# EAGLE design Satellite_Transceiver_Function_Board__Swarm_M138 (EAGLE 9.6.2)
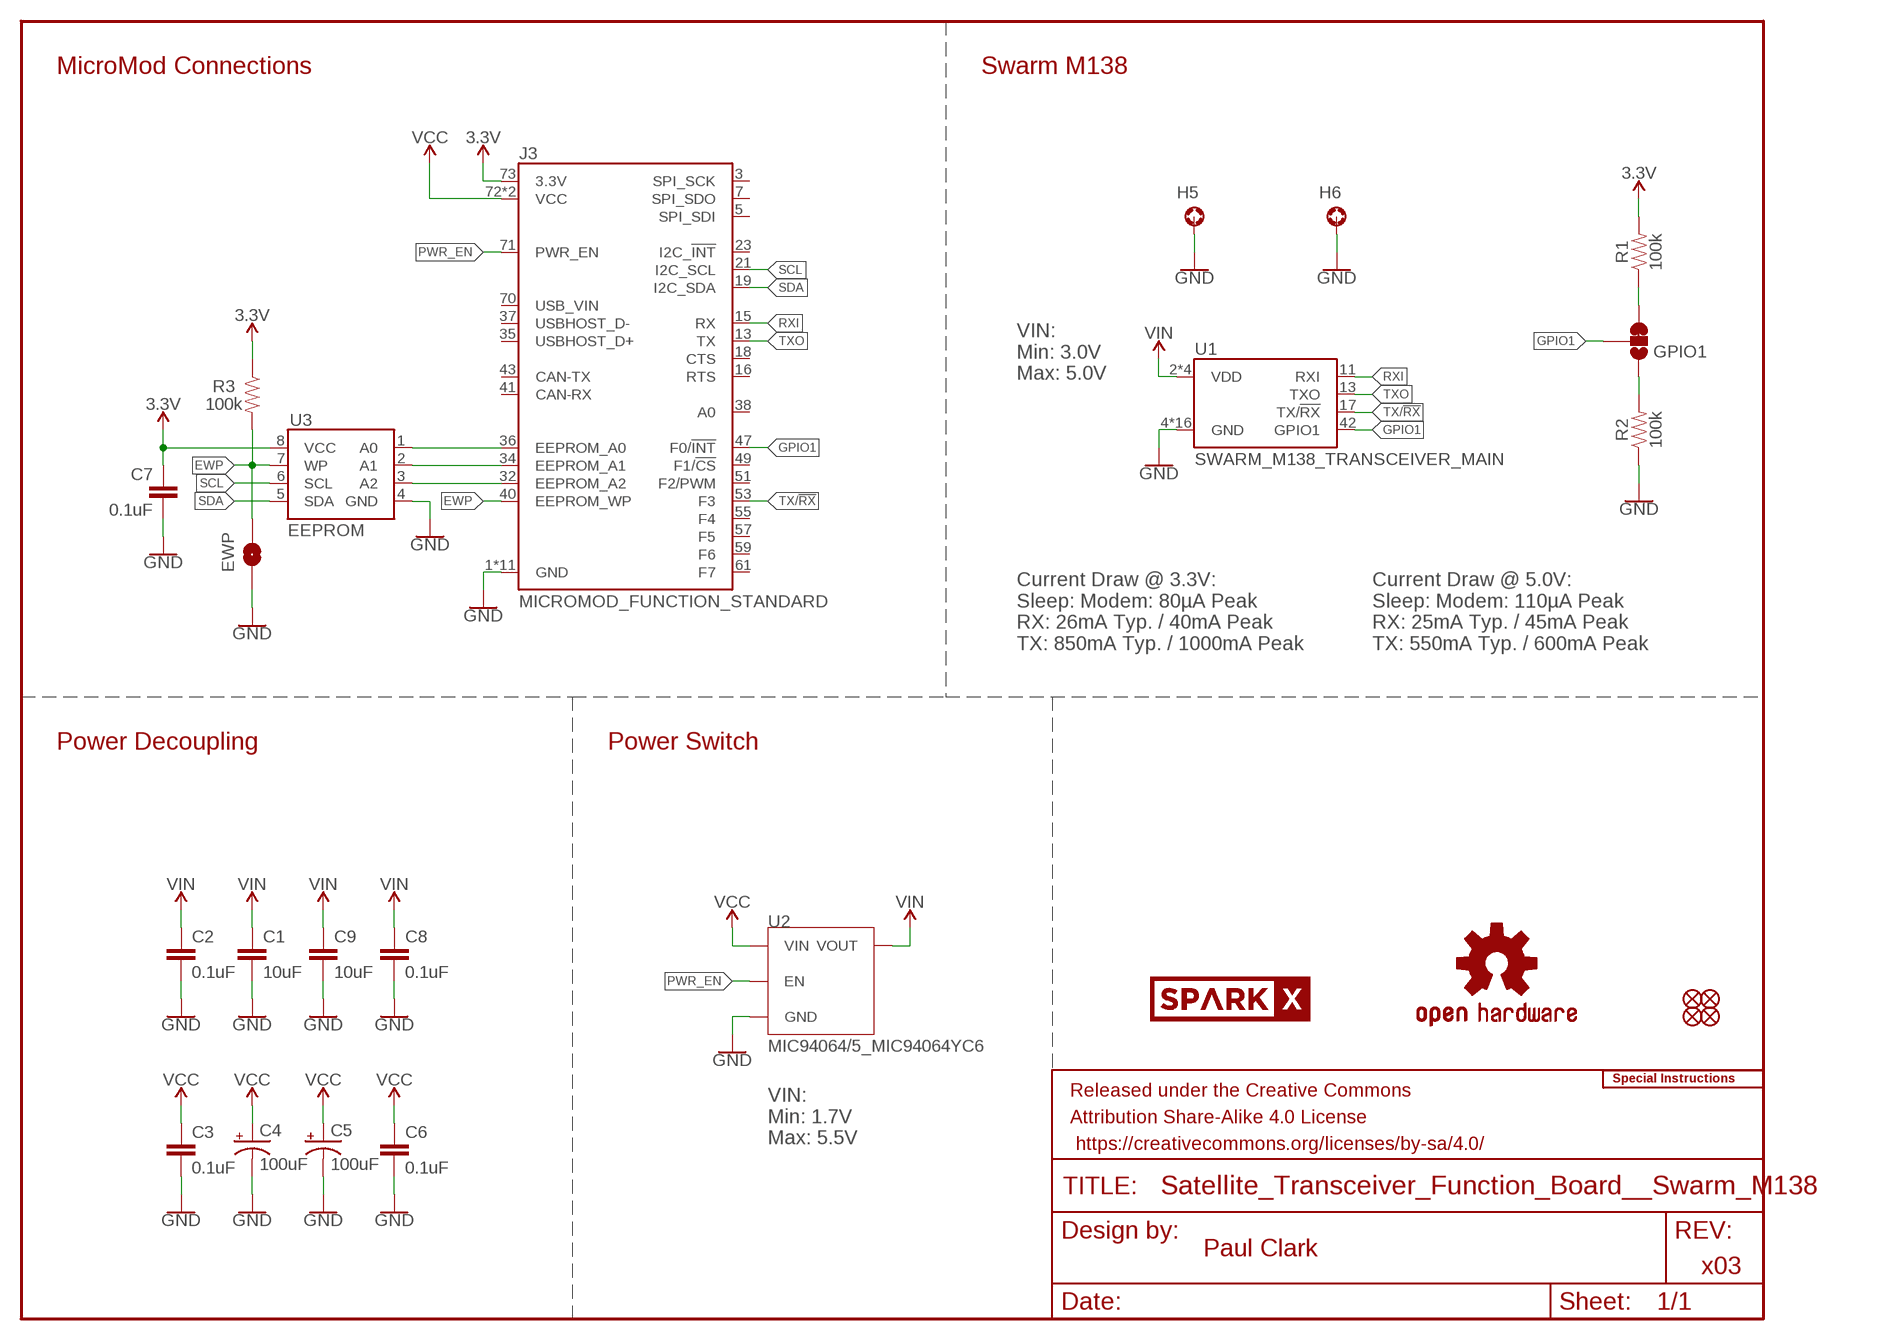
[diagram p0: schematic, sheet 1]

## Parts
C1  10uF  10UF-0603-6.3V-20%  [0603]
C2  0.1uF  0.1UF-0603-25V-5%  [0603]
C3  0.1uF  0.1UF-0603-25V-5%  [0603]
C4  100uF  100UF-POLAR-EIA3528-10V-20%(TANT)  [EIA3528]
C5  100uF  100UF-POLAR-EIA3528-10V-20%(TANT)  [EIA3528]
C6  0.1uF  0.1UF-0603-25V-5%  [0603]
C7  0.1uF  0.1UF-0603-25V-5%  [0603]
C8  0.1uF  0.1UF-0603-25V-5%  [0603]
C9  10uF  10UF-0603-6.3V-20%  [0603]
EWP  JUMPER-SMT_2_NO_SILK  [SMT-JUMPER_2_NO_SILK]
FD1  FIDUCIAL1X2  [FIDUCIAL-1X2]
FD2  FIDUCIAL1X2  [FIDUCIAL-1X2]
FD3  FIDUCIAL1X2  [FIDUCIAL-1X2]
FD4  FIDUCIAL1X2  [FIDUCIAL-1X2]
FRAME1  FRAME-LETTER  [CREATIVE_COMMONS]
GPIO1  JUMPER-SMT_3_1-NC_TRACE_SILK  [SMT-JUMPER_3_1-NC_TRACE_SILK]
H5  STAND-OFF-REFLOW-M2.5_1.5MM_TALL  [STAND-OFF-REFLOW-M2.5]
H6  STAND-OFF-REFLOW-M2.5_1.5MM_TALL  [STAND-OFF-REFLOW-M2.5]
J3  MICROMOD_FUNCTION_STANDARD  [M.2-CARD-E-22_FUNCTION_STANDARD]
LOGO1  SPECIAL_INSTRUCTIONS-ORDERING  [ORDERING_INSTRUCTIONS]
LOGO2  OSHW-LOGOM  [OSHW-LOGO-M]
LOGO3  OSHW-LOGOM  [OSHW-LOGO-M]
R1  100k  100KOHM-0603-1/10W-1%  [0603]
R2  100k  100KOHM-0603-1/10W-1%  [0603]
R3  100k  100KOHM-0603-1/10W-1%  [0603]
U1  SWARM_M138_TRANSCEIVER_MAIN  [M.2-SWARM-M138-A]
U2  MIC94064/5_MIC94064YC6  [SC-70-6]
U3  EEPROM  EEPROM-I2C512K  [SO08]
U$1  SPARKX-LOGO5  [SPARKX-LARGE]
U$2  SPARKX-LOGO5  [SPARKX-LARGE]

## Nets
3.3V: C7.1 J3.73(3.3V) R1.2 R3.1 U3.8(VCC)
A0 [DIGITAL]: J3.36(EEPROM_A0) U3.1(A0)
A1 [DIGITAL]: J3.34(EEPROM_A1) U3.2(A1)
A2 [DIGITAL]: J3.32(EEPROM_A2) U3.3(A2)
EWP [DIGITAL]: EWP.2 J3.40(EEPROM_WP) R3.2 U3.7(WP)
GND: C1.2 C2.2 C3.2 C4.C(-) C5.C(-) C6.2 C7.2 C8.2 C9.2 EWP.1 H5.1 H6.1 J3.1(GND) J3.33(GND) J3.39(GND) J3.45(GND) J3.75(GND) J3.GND1(GND) J3.GND2(GND) J3.GND3(GND) J3.GND4(GND) J3.GND5(GND) J3.GND6(GND) R2.1 U1.4(GND) U1.9(GND) U1.15(GND) U1.18(GND) U1.21(GND) U1.26(GND) U1.27(GND) U1.29(GND) U1.34(GND) U1.35(GND) U1.37(GND) U1.40(GND) U1.43(GND) U1.50(GND) U1.A1(GND) U1.A2(GND) U2.2(GND) U2.5(GND) U3.4(GND)
GPIO1: GPIO1.2 J3.47(F0/!INT!) U1.42(GPIO1)
N$14: GPIO1.3 R1.1
N$16: GPIO1.1 R2.2
PWR_EN: J3.71(PWR_EN) U2.3(EN)
RXI: J3.15(RX) U1.11(RXI)
SCL [DIGITAL]: J3.21(I2C_SCL) U3.6(SCL)
SDA [DIGITAL]: J3.19(I2C_SDA) U3.5(SDA)
TX/!RX!: J3.53(F3) U1.17(TX/!RX!)
TXO: J3.13(TX) U1.13(TXO)
VCC: C3.1 C4.A(+) C5.A(+) C6.1 J3.72(VCC) J3.74(VCC) U2.4(VIN)
VIN: C1.1 C2.1 C8.1 C9.1 U1.2(VDD) U1.39(VDD) U1.41(VDD) U1.52(VDD) U2.1(VOUT)
Unconnected: J3.3(SPI_SCK) J3.5(SPI_SDI) J3.7(SPI_SDO) J3.16(RTS) J3.18(CTS) J3.23(I2C_!INT!) J3.35(USBHOST_D+) J3.37(USBHOST_D-) J3.38(A0) J3.41(CAN-RX) J3.43(CAN-TX) J3.49(F1/!CS!) J3.51(F2/PWM) J3.55(F4) J3.57(F5) J3.59(F6) J3.61(F7) J3.70(USB_VIN)

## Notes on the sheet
- MicroMod Connections | Swarm M138
- VIN:
  Min: 3.0V
  Max: 5.0V
- Current Draw @ 3.3V:
  Sleep: Modem: 80µA Peak
  RX: 26mA Typ. / 40mA Peak
  TX: 850mA Typ. / 1000mA Peak
- Current Draw @ 5.0V:
  Sleep: Modem: 110µA Peak
  RX: 25mA Typ. / 45mA Peak
  TX: 550mA Typ. / 600mA Peak
- Power Decoupling | Power Switch
- VIN:
  Min: 1.7V
  Max: 5.5V
- Paul Clark
- x03

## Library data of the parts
C1 C9 = SparkFun-Capacitors:10UF: 10.0µF ceramic capacitors; PROD_ID: CAP-11015
C2 C3 C6-C8 = SparkFun-Capacitors:0.1UF: 0.1µF ceramic capacitors; PROD_ID: CAP-08604
C4 C5 = SparkFun-Capacitors:100UF-POLAR: 100µF polarized capacitors; PROD_ID: CAP-16823
EWP = SparkFun-Jumpers:JUMPER-SMT_2_NO: Normally open jumper
FD1-FD4 = SparkFun-Aesthetics:FIDUCIAL: Fiducial Alignment Points
FRAME1 = SparkFun-Aesthetics:FRAME-LETTER: Schematic Frame - Letter
GPIO1 = SparkFun-Jumpers:JUMPER-SMT_3_1-NC_TRACE: Normally closed trace jumper (1 of 2 connections) This jumper has a trace between two pads so it's normally closed (NC). The other connection is normally open (NO). Use a razor knife to open the connection. For best results follow the IPC guidelines for cutting traces: Cutout at least 0.063 mm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
H5 H6 = SparkFun-Hardware:STAND-OFF-REFLOW: Stand Off Reflow Compatible; PROD_ID: HW-16629
J3 = SparkFun-MicroMod:MICROMOD_FUNCTION: MicroMod Connector Description: A card edge connector and mating PCB connector to allow various MicroMod Processor Boards to be coupled with various carrier boards of different capabilities. Based on the M.2 standard.
LOGO1 = SparkFun-Aesthetics:SPECIAL_INSTRUCTIONS: Special Ordering/Production Instructions Alert
LOGO2 LOGO3 = SparkFun-Aesthetics:OSHW-LOGO: Open-Source Hardware (OSHW) Logo
R1-R3 = SparkFun-Resistors:100KOHM: 100kΩ resistor; PROD_ID: RES-07828
U1 = SparkFun-RF:SWARM_M138_TRANSCEIVER: Swarm M138 Modem Description: A satellite transceiver based on the mPCIe standard.; PROD_ID: CONN-16558
U2 = SparkFun-IC-Power:MIC94064/5: The MIC94064 and MIC94065 are high-side load switches designed for operation between 1.7V to 5.5V. The devices contain a low on-resistance P-channel MOSFET that supports over 2A of continuous current. The MIC94064/5 provides a slew rate controlled SoftStart turn-on of 115µs (typical) to prevent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; PROD_ID: IC-16794
U3 = SparkFun-IC-Memory:EEPROM-I2C: I2C EEPROMs, 24LC256 and others 24LC256 Series 256 kb I2C 2 Wire (32 k x 8 Bit) 2.5 V Serial EEPROM SMD - SOIC-8 Datasheet SparkFun Products SparkFun UDB5 - PIC UAV Development Board (GPS-11703); PROD_ID: IC-14645
U$1 U$2 = SparkX:SPARKX-LOGO

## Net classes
4 3.3V: width 0.2 mm, clearance 0.2 mm to class 1
10 DIGITAL: width 0.09 mm, clearance 0.1 mm to class 0, clearance 0.1 mm to class 1, clearance 0.1 mm

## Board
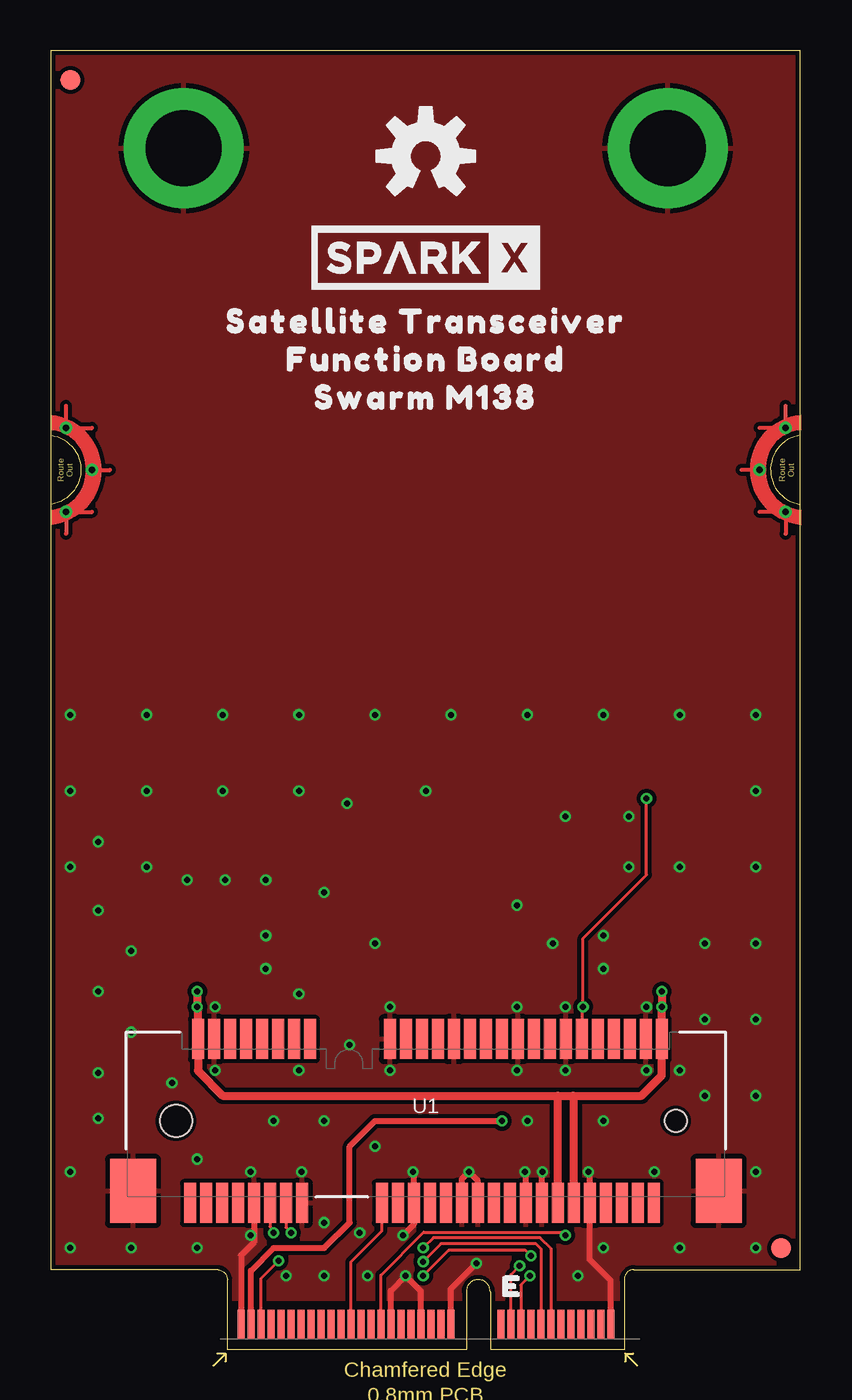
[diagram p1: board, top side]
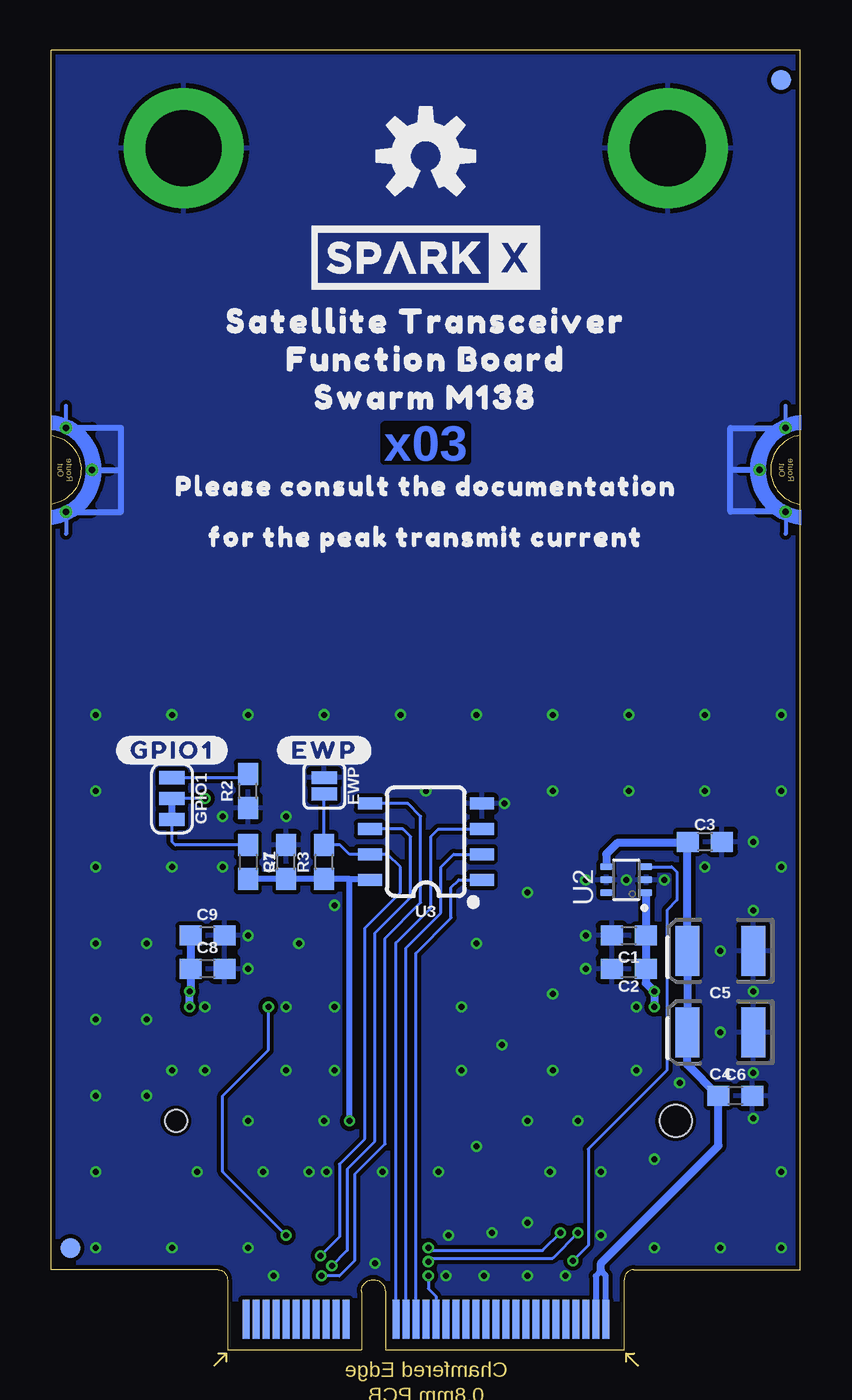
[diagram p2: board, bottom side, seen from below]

Size 37.5 x 65 mm. Coordinates in mm from the lower left corner, seen from the top.
Outline: 28.67,0 21.97,0 21.97,2.9 arc180 20.77,2.9 20.77,0 8.82,0 8.82,3.5 arc84 8.35,4 0,4 0,65 37.49,65 37.49,4 29.15,4 arc85 28.67,3.5 28.67,0
Copper layers (1*16): Top 0.035mm / dielectric 1.5mm / Bottom 0.035mm
Design rules "SparkFun-2-Layer-Minimum-JLCPCB": minimum track width 5mil, minimum drill 0.3mm, track to track 5mil, track to pad 5mil, pad to pad 5mil, via to via 5mil, smd to smd 5mil, copper to edge 7mil, drill to drill 7mil, minimum pad ring 5mil, minimum via ring 5mil, stop-mask expansion 2.5mil, vias tented up to drill 25mil, thermal gap 10mil
tRestrict: 2 lines

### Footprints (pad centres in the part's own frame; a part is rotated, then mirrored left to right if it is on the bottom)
0603 = smd 1.1 x 1: 1 -0.85,0; 2 0.85,0
EIA3528 = smd 1.2 x 2.5: A 1.65,0; C -1.65,0
SMT-JUMPER_2_NO_SILK = smd 0.635 x 1.27: 1 -0.406,0; 2 0.406,0
FIDUCIAL-1X2 = smd 1 x 1: 1 0,0
SMT-JUMPER_3_1-NC_TRACE_SILK = smd 0.66 x 1.27: 1 -1.041,0; 2 0,0; 3 1.041,0
STAND-OFF-REFLOW-M2.5 = drill 3.8 pad 6: 1 0,0
M.2-CARD-E-22_FUNCTION_STANDARD = smd 0.35 x 1.45: 1 9.25,1.275; 3 8.75,1.275; 5 8.25,1.275; 7 7.75,1.275; 9 7.25,1.275; 11 6.75,1.275; 13 6.25,1.275; 15 5.75,1.275; 17 5.25,1.275; 19 4.75,1.275; 21 4.25,1.275; 23 3.75,1.275; 33 1.25,1.275; 35 0.75,1.275; 37 0.25,1.275; 39 -0.25,1.275; 41 -0.75,1.275; 43 -1.25,1.275; 45 -1.75,1.275; 47 -2.25,1.275; 49 -2.75,1.275; 51 -3.25,1.275; 53 -3.75,1.275; 55 -4.25,1.275; 57 -4.75,1.275; 59 -5.25,1.275; 61 -5.75,1.275; 63 -6.25,1.275; 65 -6.75,1.275; 67 -7.25,1.275; 69 -7.75,1.275; 71 -8.25,1.275; 73 -8.75,1.275; 75 -9.25,1.275 | smd 0.35 x 1.95 bottom: 2 9,1.525; 4 8.5,1.525; 6 8,1.525; 8 7.5,1.525; 10 7,1.525; 12 6.5,1.525; 14 6,1.525; 16 5.5,1.525; 18 5,1.525; 20 4.5,1.525; 22 4,1.525; 32 1.5,1.525; 34 1,1.525; 36 0.5,1.525; 38 0,1.525; 40 -0.5,1.525; 42 -1,1.525; 44 -1.5,1.525; 46 -2,1.525; 48 -2.5,1.525; 50 -3,1.525; 52 -3.5,1.525; 54 -4,1.525; 56 -4.5,1.525; 58 -5,1.525; 60 -5.5,1.525; 62 -6,1.525; 64 -6.5,1.525; 66 -7,1.525; 68 -7.5,1.525; 70 -8,1.525; 72 -8.5,1.525; 74 -9,1.525 | drill 0.305 pad 0.61: GND1 -18,41.9; GND2 -16.7,44; GND3 -18,46.1; GND4 18,41.9; GND5 16.7,44; GND6 18,46.1
M.2-SWARM-M138-A = smd 0.6 x 2: 1 -11.8,-4.1; 2 -11.4,4.1; 3 -11,-4.1; 4 -10.6,4.1; 5 -10.2,-4.1; 6 -9.8,4.1; 7 -9.4,-4.1; 8 -9,4.1; 9 -8.6,-4.1; 10 -8.2,4.1; 11 -7.8,-4.1; 12 -7.4,4.1; 13 -7,-4.1; 14 -6.6,4.1; 15 -6.2,-4.1; 16 -5.8,4.1; 17 -2.2,-4.1; 18 -1.8,4.1; 19 -1.4,-4.1; 20 -1,4.1; 21 -0.6,-4.1; 22 -0.2,4.1; 23 0.2,-4.1; 24 0.6,4.1; 25 1,-4.1; 26 1.4,4.1; 27 1.8,-4.1; 28 2.2,4.1; 29 2.6,-4.1; 30 3,4.1; 31 3.4,-4.1; 32 3.8,4.1; 33 4.2,-4.1; 34 4.6,4.1; 35 5,-4.1; 36 5.4,4.1; 37 5.8,-4.1; 38 6.2,4.1; 39 6.6,-4.1; 40 7,4.1; 41 7.4,-4.1; 42 7.8,4.1; 43 8.2,-4.1; 44 8.6,4.1; 45 9,-4.1; 46 9.4,4.1; 47 9.8,-4.1; 48 10.2,4.1; 49 10.6,-4.1; 50 11,4.1; 51 11.4,-4.1; 52 11.8,4.1 | smd 2.3 x 3.2: A1 -14.65,-3.5; A2 14.65,-3.5 | hole 1.1: 12.5,0 | hole 1.6: -12.5,0
SC-70-6 = smd 0.35 x 0.6: 1 -0.65,-1; 2 0,-1; 3 0.65,-1; 4 0.65,1; 5 0,1; 6 -0.65,1
SO08 = smd 0.6 x 1.2: 1 -1.905,-2.8; 2 -0.635,-2.8; 3 0.635,-2.8; 4 1.905,-2.8; 5 1.905,2.8; 6 0.635,2.8; 7 -0.635,2.8; 8 -1.905,2.8

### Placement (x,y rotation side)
C1  8.59,20.7 180 bottom
C2  8.59,19.05 180 bottom
C3  4.78,25.4 0 bottom
C4  4.02,15.88 180 bottom
C5  4.02,19.94 180 bottom
C6  3.25,12.7 0 bottom
C7  25.73,24.38 90 bottom
C8  29.67,19.05 0 bottom
C9  29.67,20.7 0 bottom
EWP  23.83,28.19 270 bottom
FD1  36.53,5.08 0 top
FD2  36.53,5.08 0 bottom
FD3  0.97,63.5 0 top
FD4  0.97,63.5 0 bottom
FRAME1  not placed on the board
GPIO1  31.45,27.56 270 bottom
H5  6.65,60.08 0 top
H6  30.85,60.08 0 top
J3  18.75,0 0 top
LOGO1  not placed on the board
LOGO2  18.75,59.69 0 top
LOGO3  18.75,59.69 0 bottom
R1  27.64,24.38 270 bottom
R2  27.64,27.94 90 bottom
R3  23.83,24.38 90 bottom
U1  18.75,11.43 0 top
U2  8.71,23.5 90 bottom
U3  18.75,25.4 90 bottom
U$1  18.75,54.61 0 bottom
U$2  18.75,54.61 0 top
U$3  [FUNCTION_BOARD0]  18.75,49.53 0 top
U$4  [SATELLITE_TRANSCEIVER0]  18.75,51.44 0 top
U$5  [SATELLITE_TRANSCEIVER0]  18.75,51.44 0 bottom
U$6  [PLEASE_CONSULT_THE_DOCUMENTATION0]  18.75,43.18 0 bottom
U$7  [FUNCTION_BOARD0]  18.75,49.53 0 bottom
U$8  [#EWP#0]  23.83,29.97 0 bottom
U$19  [#GPIO1#0]  31.45,29.97 0 bottom
U$31  [FOR_THE_PEAK_TRANSMIT_CURRENT1]  18.75,40.64 0 bottom
U$40  [SWARM_M1381]  18.75,47.62 0 top
U$41  [SWARM_M1381]  18.75,47.62 0 bottom

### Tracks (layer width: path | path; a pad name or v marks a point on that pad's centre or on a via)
3.3V  (via drill 0.3)
  Top 0.305: J3.73 10,3.95 11.13,5.08 13.67,5.08 14.94,6.35 14.94,10.16 16.21,11.43 v22.56,11.43
  Bottom 0.305: v22.56,11.43 22.56,23.53 | 22.56,23.53 R3.1 C7.1 R1.2 | 22.56,23.53 21.59,23.53 U3.8
A0
  Bottom 0.152: U3.1 17.1,23.5 17.48,23.11 17.48,21.59 19.25,19.82 J3.36
A1
  Bottom 0.152: U3.2 17.35,24.77 17.98,24.13 17.98,21.84 19.75,20.08 J3.34
A2
  Bottom 0.152: J3.32 20.25,20.34 18.49,22.1 18.49,25.65 18.11,26.04 U3.3
EWP  (via drill 0.3)
  Top 0.152: v24.02,4.68 23.75,4.95 19.89,4.95 v18.62,3.68
  Bottom 0.152: v24.02,4.68 23.06,5.63 23.06,9.27 21.8,10.54 21.8,21.08 20.02,22.86 20.02,24.13 20.65,24.77 U3.7 22.56,24.77 23.03,25.23 R3.2 EWP.2 | v18.62,3.68 18.62,3.05 18.25,2.67 J3.40
GND  (via drill 0.3)
  Top 0.305: J3.1 28,3.45 26.95,4.5 U1.43 26.95,8.82 v26.88,8.89 | U1.9 10.15,5.37 9.5,4.72 J3.75 | J3.33 20,3.03 v21.29,4.32 | U1.27 20.55,8.53 v20.91,8.89 21.35,8.45 U1.29 | v18.11,8.89 18.15,8.86 U1.21 18.15,6.26 v17.6,5.71 | U1.35 23.75,8.84 v23.7,8.89 | U1.37 24.55,8.85 v24.59,8.89 | J3.39 18.5,2.92 v17.73,3.68 17,2.95 J3.45
  Bottom 0.305: J3.GND1 3.51,41.91 3.51,44 | J3.GND3 3.51,46.1 3.51,44 | J3.GND2 3.51,44 | J3.GND5 33.99,44 | J3.GND6 33.99,46.1 33.99,44 | J3.GND4 33.99,41.9 33.99,44
  other vias: 16.97,13.97 23.32,13.97 25.73,13.97 29.8,13.97 2.36,25.4 9.98,8.89 8.21,13.97 12.52,8.89 27.64,19.05 25.73,17.14 23.32,17.14 16.97,17.14 29.8,17.14 31.45,13.97 27.64,11.43 16.21,10.16 13.67,11.43 13.67,6.35 15.45,5.84 13.67,3.68 26.37,3.68 7.32,5.08 0.97,5.08 2.36,17.91 2.36,21.97 0.97,31.75 4.78,31.75 8.59,31.75 12.4,31.75 16.21,31.75 20.02,31.75 23.83,31.75 35.26,31.75 8.59,27.94 12.4,27.94 31.45,31.75 35.26,24.13 27.64,31.75 8.21,17.14 12.4,17.78 12.4,13.97 2.36,13.84 11.13,11.43 30.18,8.89 31.45,5.08 35.26,27.94 2.36,11.56 4.02,5.08 15.83,3.68 9.98,5.71 23.83,11.43 11.76,3.68 35.26,5.08 8.71,23.5 6.81,23.5 10.75,23.5 7.32,9.53 6.05,13.34 0.97,8.89 4.02,19.94 4.02,15.88 10.75,20.7 10.75,19.05 4.78,27.94 0.97,27.94 27.64,20.7 14.81,27.3 25.73,26.67 0.97,24.13 4.78,24.13 31.45,24.13 35.26,20.32 35.26,16.51 35.26,12.7 35.26,8.89 32.72,20.32 32.72,16.51 32.72,12.7 25.1,20.32 16.21,20.32 14.94,15.24 13.67,22.86 23.32,22.23 18.75,27.94 27.64,5.08 28.91,24.13 28.91,26.67
  pour Top (isolate 0.203): -0.3,2.54 -0.3,66.04 37.8,66.04 37.8,2.54
  pour Bottom (isolate 0.203): -0.3,2.54 -0.3,66.04 37.8,66.04 37.8,2.54
GPIO1  (via drill 0.3)
  Top 0.152: J3.47 16.5,3.72 18.64,5.87 25.58,5.87 v25.73,5.71 | U1.42 26.55,17.07 v26.62,17.14 26.62,20.57 29.8,23.75 v29.8,27.56
  Bottom 0.152: v25.73,5.71 28.91,8.89 28.91,12.7 26.62,14.99 v26.62,17.14 | v29.8,27.56 GPIO1.2
N$14
  Bottom 0.152: R1.1 31.28,25.23 31.45,25.4 GPIO1.3
N$16
  Bottom 0.152: GPIO1.1 27.83,28.6 R2.2
PWR_EN  (via drill 0.3)
  Top 0.152: J3.71 10.5,3.56 v11.38,4.45
  Bottom 0.152: U2.3 6.44,24.14 6.17,23.88 6.17,22.48 6.68,21.97 6.68,13.97 10.62,10.03 10.62,5.21 v11.38,4.45
RXI  (via drill 0.3)
  Top 0.152: U1.11 10.95,6.15 11.13,5.97 v11.13,5.84 | v18.62,4.4 19.51,5.29 24.25,5.29 24.5,5.04 J3.15
  Bottom 0.152: v11.13,5.84 12.4,4.57 18.45,4.57 v18.62,4.4
SCL  (via drill 0.3)
  Top 0.152: J3.21 23,3.74 v23.45,4.19
  Bottom 0.152: v23.45,4.19 22.68,4.95 22.68,9.02 21.29,10.41 21.29,20.83 19.51,22.61 19.51,25.65 19.89,26.04 U3.6
SDA  (via drill 0.3)
  Top 0.152: v23.95,3.68 23.5,3.23 J3.19
  Bottom 0.152: v23.95,3.68 23.06,3.68 22.3,4.45 22.3,8.76 20.78,10.29 20.78,20.57 19,22.35 19,26.67 19.64,27.3 U3.5
TX/!RX!
  Top 0.152: J3.53 15,4.38 16.55,5.93 U1.17
TXO  (via drill 0.3)
  Top 0.152: U1.13 11.75,6.11 v12.02,5.84 | J3.13 25,5.05 24.46,5.59 19.13,5.59 v18.62,5.08
  Bottom 0.152: v18.62,5.08 18.49,4.95 12.91,4.95 v12.02,5.84
VCC
  Bottom 0.305: J3.74 9.75,3.7 9.98,3.94 10.25,3.67 J3.72 | 9.71,24.24 U2.4
  Bottom 0.406: 9.98,3.94 9.98,4.32 4.1,10.2 C6.1 5.66,14.26 C4.A C5.A 5.66,25.36 | 9.71,24.24 9.71,24.78 9.13,25.36 5.66,25.36 | 5.66,25.36 C3.1
VIN  (via drill 0.3)
  Top 0.406: 25.35,12.7 8.59,12.7 7.35,13.94 U1.2 7.35,17.11 v7.32,17.14 v7.32,17.91 | 25.35,12.7 26.11,12.7 | 26.11,12.7 29.54,12.7 30.55,13.71 U1.52 v30.55,17.13 v30.56,17.14 v30.56,17.91 | U1.39 25.35,12.7 | U1.41 26.15,12.67 26.11,12.7
  Bottom 0.305: 7.71,22.62 U2.1
  Bottom 0.406: v7.32,17.14 v7.32,17.91 7.74,18.33 C2.1 C1.1 7.71,20.72 7.71,22.62 | v30.56,17.14 v30.56,17.91 30.52,17.95 C8.1 C9.1

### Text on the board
Bottom: x03
Measures: Dimensions in mm
tDocu: 2-Layer Board / 0.8mm Thickness / 1oz Copper / ENIG Finish / Chamfered Edge | Paul Clark

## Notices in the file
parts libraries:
SparkFun-Aesthetics: Licensing: Creative Commons ShareAlike 4.0 International - https://creativecommons.org/licenses/by-sa/4.0
SparkFun-Aesthetics: Released under the Creative Commons Attribution Share-Alike 4.0 License
SparkFun-Aesthetics: https://creativecommons.org/licenses/by-sa/4.0
